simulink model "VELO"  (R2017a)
settings: Solver=VariableStepAuto  StartTime=0.0  StopTime=120  RelTol=1e-3  EnableMultiTasking=on
undefined symbols (not defined in the file): sigbuilder_block
libraries: fl_lib x16, nesl_utility x7, elec_lib x2, sdl_lib x1

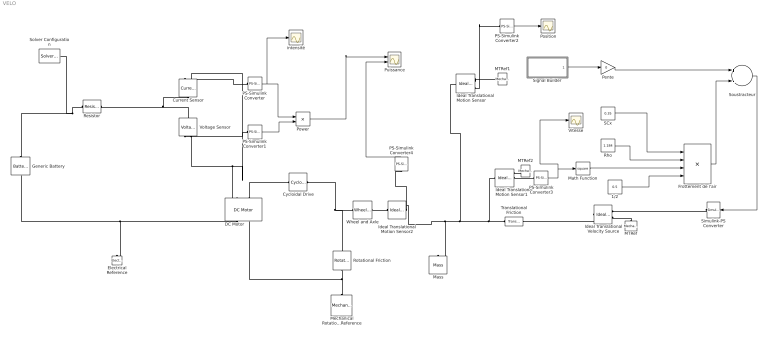
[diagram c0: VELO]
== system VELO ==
  1/2 : Constant  Value=0.5
  Current Sensor : fl_lib/Electrical/Electrical Sensors/Current Sensor
  Cycloidal Drive : sdl_lib/Gears/Cycloidal Drive  n_cycloid=20  n_ring=24  eff_BF=0.90  eff_FB=0.05  pwr_thr=0.001 W  temperature_TLU=[280, 300, 320] K  efficiency_BF_TLU=[.95, .85, .80]  efficiency_FB_TLU=[.10, .05, .03]  thermal_mass=50 J/K  T_init=300 K
  DC Motor : elec_lib/Actuators & Drivers/Rotational Actuators/DC Motor  parameterization=1  Ra=3.9 Ohm  La=1.2e-5 H  emf_or_torque=1  Kv=7.2e-5 V/rpm  Ki=6.876e-4 N*m/A  T_stall=2.4e-4 N*m  w_max=1.91e+4 rpm  w_rated=1.5e+4 rpm  P_rated=0.08 W  V_rated=1.5 V  J=0.01 g*cm^2  lam_param=1  lam=0 N*m/(rad/s)  i_noload=0 A  V_i_noload=1.5 V  speed0=0 rpm  alpha=0.00393 1/K  Tmeas=25 C  thermal_mass=100 J/K  initial_temperature=25 C
  Electrical Reference : fl_lib/Electrical/Electrical Elements/Electrical Reference
  Frottement de l'air : Product  Inputs=4
  Generic Battery : elec_lib/Sources/Battery  Vnom=24 V  R1=12 Ohm  prm_AH=2  AH=8 hr*A  V1=11.5 V  AH1=2 hr*A  prm_R2=1  R2=2e+3 Ohm  prm_fade=1  N_fade=100  AH_fade=45 hr*A  R1_fade=2.02 Ohm  V1_fade=10.35 V  i_specify=off  i_priority=None  i=0 A  i_nominal_specify=off  i_nominal_unit=A  i_nominal_value=1  v_specify=off  v_priority=None  v=0 V  v_nominal_specify=off  v_nominal_unit=V  v_nominal_value=1  charge_specify=on  charge_priority=High  charge=50 hr*A  charge_nominal_specify=off  charge_nominal_unit=hr*A  charge_nominal_value=1  num_cycles_specify=off  num_cycles_priority=High  num_cycles=0  num_cycles_nominal_specify=off  num_cycles_nominal_unit=1  num_cycles_nominal_value=1  thermal_mass=30000 J/K  Tmeas=298.15 K  Vnom_T2=12 V  R1_T2=2.2 Ohm  V1_T2=11.4 V  R2_T2=2200 Ohm  Tmeas2=273.15 K  temperature_specify=off  temperature_priority=High  temperature=298.15 K  temperature_nominal_specify=off  temperature_nominal_unit=K  temperature_nominal_value=1
  Ideal Translational Motion Sensor : fl_lib/Mechanical/Mechanical Sensors/Ideal Translational Motion Sensor  offset=0 m
  Ideal Translational Motion Sensor1 : fl_lib/Mechanical/Mechanical Sensors/Ideal Translational Motion Sensor  offset=0 m
  Ideal Translational Motion Sensor2 : fl_lib/Mechanical/Mechanical Sensors/Ideal Translational Motion Sensor  offset=0 m
  Ideal Translational Velocity Source : fl_lib/Mechanical/Mechanical Sources/Ideal Translational Velocity Source
  MTRef : fl_lib/Mechanical/Translational Elements/Mechanical Translational Reference  Tag=Factory Generic
  MTRef1 : fl_lib/Mechanical/Translational Elements/Mechanical Translational Reference  Tag=Factory Generic
  MTRef2 : fl_lib/Mechanical/Translational Elements/Mechanical Translational Reference  Tag=Factory Generic
  Mass : fl_lib/Mechanical/Translational Elements/Mass  mass=93.5 kg  v_specify=off  v_priority=None  v=0 m/s  v_nominal_specify=off  v_nominal_unit=m/s  v_nominal_value=1  f_specify=off  f_priority=None  f=0 N  f_nominal_specify=off  f_nominal_unit=N  f_nominal_value=1
  Math Function : Math  Operator=square
  Mechanical Rotational Reference : fl_lib/Mechanical/Rotational Elements/Mechanical Rotational Reference
  PS-Simulink Converter{,1..4} (5 alike) : nesl_utility/PS-Simulink Converter  PhysicalDomain=network_engine_domain  SubClassName=ps_output  LeftPortType=input  RightPortType=output  PseudoPeriodic=off  Frequencies=[]  Unit=1  AffineConversion=off
  Pente : Gain  Gain=0
  Position : Scope
  Power : Product
  Puissance : Scope  NumInputPorts=2
  Resistor : fl_lib/Electrical/Electrical Elements/Resistor  R=12 Ohm  i_specify=off  i_priority=None  i=0 A  i_nominal_specify=off  i_nominal_unit=A  i_nominal_value=1  v_specify=off  v_priority=None  v=0 V  v_nominal_specify=off  v_nominal_unit=V  v_nominal_value=1
  Rho : Constant  Value=1.184
  Rotational Friction : fl_lib/Mechanical/Rotational Elements/Rotational Friction  brkwy_trq=26 N*m  brkwy_vel=0.060623 rad/s  Col_trq=20 N*m  visc_coef=0.001 N*m/(rad/s)  w_specify=off  w_priority=None  w=0 rad/s  w_nominal_specify=off  w_nominal_unit=rad/s  w_nominal_value=1  t_specify=off  t_priority=None  t=0 N*m  t_nominal_specify=off  t_nominal_unit=N*m  t_nominal_value=1
  SCx : Constant  Value=0.35
  Signal Builder : Subsystem  Tag=STV Subsys  LoadFcn=sigbuilder_block('load');  StartFcn=sigbuilder_block('start');  StopFcn=sigbuilder_block('stop');  ClipboardFcn=sigbuilder_block('clipboard');
  Simulink-PS Converter : nesl_utility/Simulink-PS Converter  PhysicalDomain=network_engine_domain  SubClassName=ps_input  LeftPortType=input  RightPortType=output  PseudoPeriodic=off  Frequencies=[]  NoiseDistribution=none  NoiseParameters=[]  Unit=1  AffineConversion=off  FilteringAndDerivatives=zero  SimscapeFilterOrder=1  InputFilterTimeConstant=0.001  UdotUserProvided=1
  Solver Configuration : nesl_utility/Solver Configuration  PhysicalDomain=network_engine_domain  SubClassName=solver  LeftPortType=input  RightPortType=generic  Accelerate=off  Tones=[]  Harmonics=[]  SimulateNoise=off  Profile=off  UseLocalSampling=off  EnableSwitchedLinearOptims=on  FrequencyDomain=off  UseCCode=off  RelTol=0.001  AbsTol=1e-06  MinStep=1e-09  ToWorkspace=off  RevertToSquareIcSolve=off  NumHomotopyIterations=100  PhasorMode=off  PhasorModeNumHarmonics=1  OverrideAbsTol=off  DoDC=off  ResidualTolerance=1e-09  UseLocalSolver=off  LocalSolverChoice=NE_BACKWARD_EULER_ADVANCER  LocalSolverSampleTime=0.001  DoFixedCost=off  MaxNonlinIter=3  MaxModeIter=2  LinearAlgebra=Sparse  DelaysMemoryBudget=1024  AutomaticFiltering=on  FilteringTimeConstant=0.001
  Soustracteur : Sum  Inputs=+-
  Translational Friction : fl_lib/Mechanical/Translational Elements/Translational Friction  brkwy_frc=25 N  brkwy_vel=0.060623 m/s  Col_frc=20 N  visc_coef=100 N/(m/s)  v_specify=off  v_priority=None  v=0 m/s  v_nominal_specify=off  v_nominal_unit=m/s  v_nominal_value=1  f_specify=off  f_priority=None  f=0 N  f_nominal_specify=off  f_nominal_unit=N  f_nominal_value=1
  Vitesse : Scope
  Voltage Sensor : fl_lib/Electrical/Electrical Sensors/Voltage Sensor
  Wheel and Axle : fl_lib/Mechanical/Mechanisms/Wheel and Axle  R=325 mm  or=1  t_specify=off  t_priority=None  t=0 N*m  t_nominal_specify=off  t_nominal_unit=N*m  t_nominal_value=1  f_specify=off  f_priority=None  f=0 N  f_nominal_specify=off  f_nominal_unit=N  f_nominal_value=1
  intensité : Scope
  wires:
  Frottement de l'air/1 -> Soustracteur/2
  SCx/1 -> Frottement de l'air/1
  Rho/1 -> Frottement de l'air/2
  PS-Simulink Converter/1 -> intensité/1, Power/1
  PS-Simulink Converter1/1 -> Power/2
  Power/1 -> Puissance/1
  PS-Simulink Converter2/1 -> Position/1
  PS-Simulink Converter3/1 -> Math Function/1, Vitesse/1
  PS-Simulink Converter4/1 -> Puissance/2
  Pente/1 -> Soustracteur/1
  Soustracteur/1 -> Simulink-PS Converter/1
  Math Function/1 -> Frottement de l'air/3
  1/2/1 -> Frottement de l'air/4
  Signal Builder/1(Signal 2) -> Pente/1
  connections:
  DC Motor/RConn1 -- Generic Battery/RConn1 -- Electrical Reference/LConn1
  Resistor/LConn1 -- Current Sensor/LConn1 -- Voltage Sensor/LConn1
  Voltage Sensor/RConn1 -- PS-Simulink Converter1/LConn1
  Voltage Sensor/RConn2 -- Current Sensor/RConn2 -- DC Motor/LConn1
  Ideal Translational Motion Sensor/RConn3 -- PS-Simulink Converter2/LConn1
  Rotational Friction/RConn1 -- DC Motor/RConn2 -- Mechanical Rotational Reference/LConn1
  DC Motor/LConn2 -- Cycloidal Drive/LConn1
  Cycloidal Drive/RConn1 -- Rotational Friction/LConn1 -- Wheel and Axle/LConn1
  Wheel and Axle/RConn1 -- Ideal Translational Motion Sensor2/LConn1
  Ideal Translational Motion Sensor1/RConn2 -- PS-Simulink Converter3/LConn1
  Ideal Translational Motion Sensor1/LConn1 -- Translational Friction/RConn1 -- Ideal Translational Motion Sensor/LConn1 -- Ideal Translational Motion Sensor2/RConn1 -- Mass/LConn1
  Ideal Translational Motion Sensor2/RConn2 -- PS-Simulink Converter4/LConn1
  Current Sensor/RConn1 -- PS-Simulink Converter/LConn1
  Ideal Translational Velocity Source/LConn1 -- Translational Friction/LConn1
  Simulink-PS Converter/RConn1 -- Ideal Translational Velocity Source/RConn1
  MTRef/LConn1 -- Ideal Translational Velocity Source/RConn2
  Generic Battery/LConn1 -- Solver Configuration/RConn1 -- Resistor/RConn1
  MTRef2/LConn1 -- Ideal Translational Motion Sensor1/RConn1
  Ideal Translational Motion Sensor/RConn1 -- MTRef1/LConn1

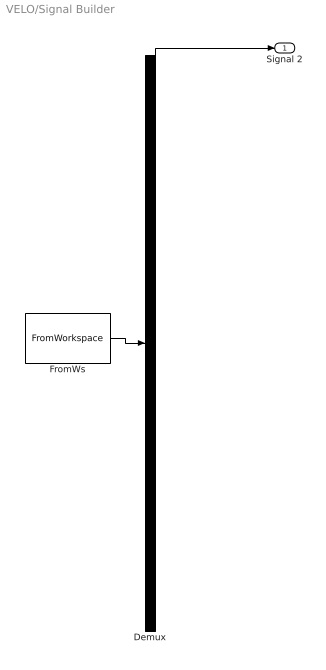
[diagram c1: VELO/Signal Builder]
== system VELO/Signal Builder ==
  Demux : Demux  Tag=STV Demux  Outputs=1
  FromWs : FromWorkspace  Tag=STV FromWs  VariableName=tuvar  SampleTime=0
  Signal 2 : Outport  Tag=STV Outport
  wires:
  FromWs/1 -> Demux/1
  Demux/1 -> Signal 2/1
